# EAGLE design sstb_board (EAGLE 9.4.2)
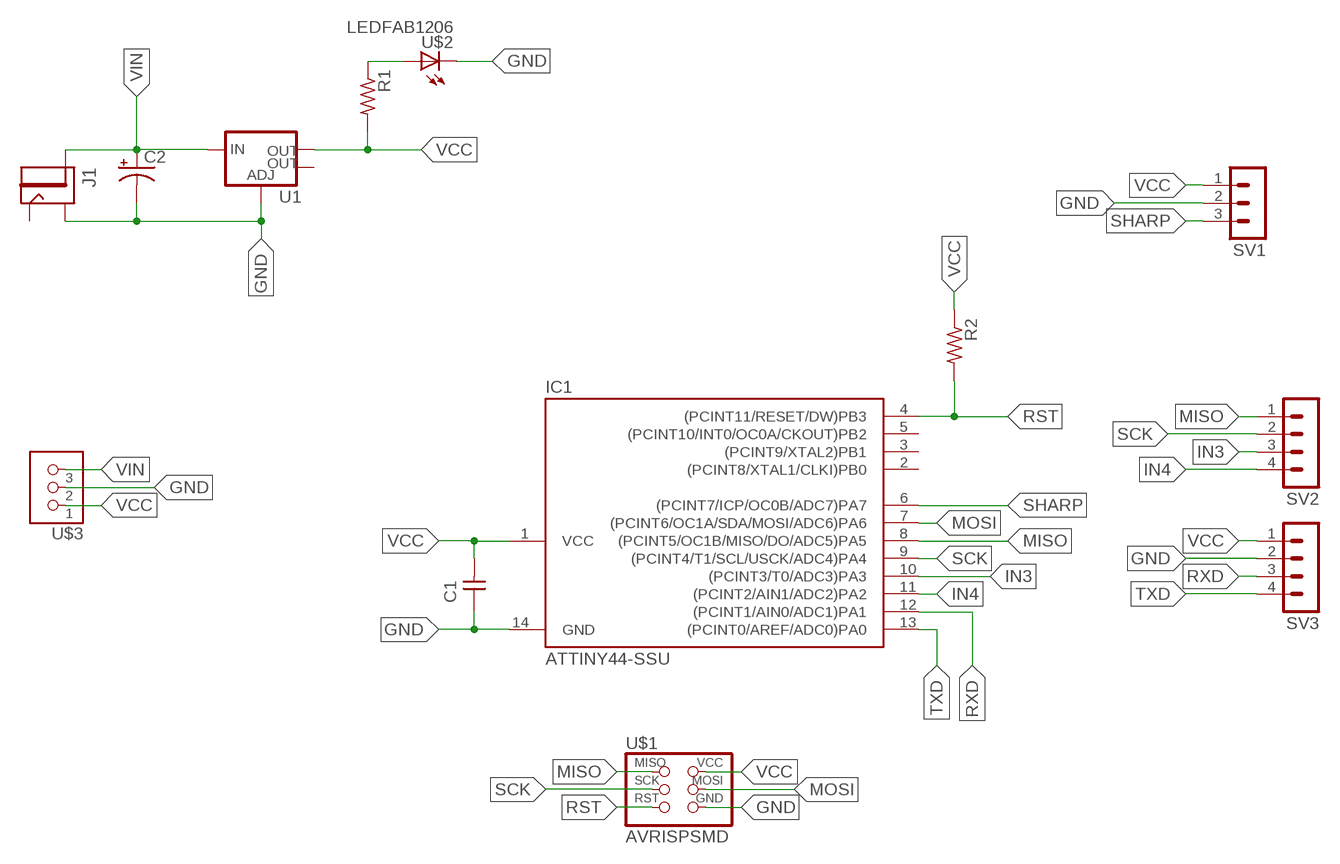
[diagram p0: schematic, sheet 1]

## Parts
C1  CAP-UNPOLARIZEDFAB  [C1206FAB]
C2  CPOL-USE5-8.5  [E5-8,5]
IC1  ATTINY44-SSU  [SOIC14]
J1  JACK2.1MM  [JACK_2.1MM]
R1  RES-US1206FAB  [R1206FAB]
R2  RES-US1206FAB  [R1206FAB]
SV1  MA03-1  [MA03-1]
SV2  MA04-1  [MA04-1]
SV3  MA04-1  [MA04-1]
U1  V_REG_LM1117SOT223  [SOT223]
U$1  AVRISPSMD  [2X03SMD]
U$2  LEDFAB1206  [LED1206FAB]
U$3  TERM-1X03'-FABLAB'  [ED555DS-3DS]

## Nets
GND: C1.1 C2.- IC1.14(GND) J1.SHUNT SV1.2 SV3.2 U1.1(ADJ) U$1.6(GND) U$2.2(C) U$3.2
IN3: IC1.10((PCINT3/T0/ADC3)PA3) SV2.3
IN4: IC1.11((PCINT2/AIN1/ADC2)PA2) SV2.4
MISO: IC1.8((PCINT5/OC1B/MISO/DO/ADC5)PA5) SV2.1 U$1.1(MISO)
MOSI: IC1.7((PCINT6/OC1A/SDA/MOSI/ADC6)PA6) U$1.4(MOSI)
N$21: R1.1 U$2.1(A)
RST: IC1.4((PCINT11/RESET/DW)PB3) R2.2 U$1.5(RST)
RXD: IC1.12((PCINT1/AIN0/ADC1)PA1) SV3.3
SCK: IC1.9((PCINT4/T1/SCL/USCK/ADC4)PA4) SV2.2 U$1.3(SCK)
SHARP: IC1.6((PCINT7/ICP/OC0B/ADC7)PA7) SV1.3
TXD: IC1.13((PCINT0/AREF/ADC0)PA0) SV3.4
VCC: C1.2 IC1.1(VCC) R1.2 R2.1 SV1.1 SV3.1 U1.2(OUT) U$1.2(VCC) U$3.1
VIN: C2.+ J1.PIN U1.3(IN) U$3.3
Unconnected: IC1.2((PCINT8/XTAL1/CLKI)PB0) IC1.3((PCINT9/XTAL2)PB1) IC1.5((PCINT10/INT0/OC0A/CKOUT)PB2) J1.CONTACT U1.4(OUT)

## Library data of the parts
C1 = fab:CAP-UNPOLARIZED
C2 = rcl:CPOL-US: POLARIZED CAPACITOR, American symbol; SPICEPREFIX: C
IC1 = fab:ATTINY44
J1 = fab:JACK
R1 R2 = fab:RES-US: Resistor (US Symbol)
SV1 = con-lstb:MA03-1: PIN HEADER; OC_FARNELL: unknown; OC_NEWARK: unknown
SV2 SV3 = con-lstb:MA04-1: PIN HEADER; OC_FARNELL: unknown; OC_NEWARK: unknown
U1 = fab:V_REG_LM1117: Voltage Regulator LM1117 Standard adjustable voltage regulator but in SMD form. Spark Fun Electronics SKU : COM-00595; PROD_ID: VREG-08170
U$1 = fab:AVRISP
U$2 = fab:LED: LED
U$3 = fab:TERM-1X03: 3.5mm terminal block, 3 positions ED555-3DS as found in the fablab inventory. Made by Zaerc.

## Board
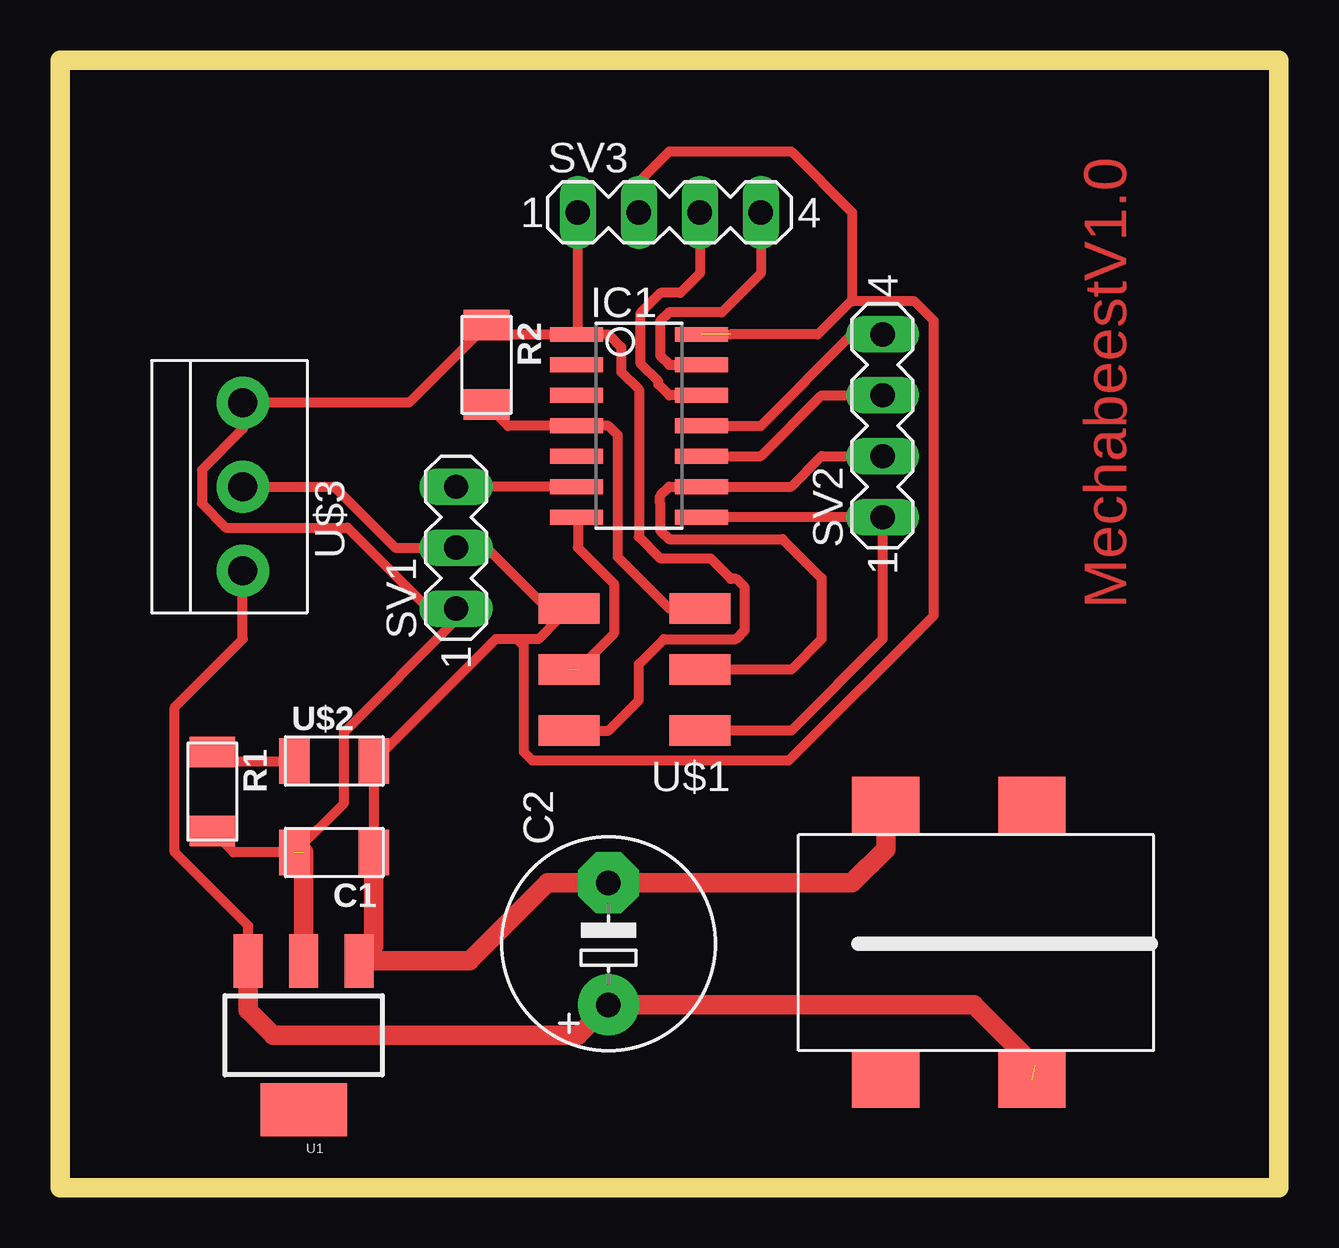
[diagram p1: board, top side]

Size 50.8 x 46.99 mm. Coordinates in mm from the lower left corner, seen from the top.
Outline: 1.27,0 2.54,0 50.8,0 50.8,46.99 0,46.99 0,0 1.27,0
Copper layers (1*16): Top 0.035mm / dielectric 1.5mm / Bottom 0.035mm
Design rules "default *": minimum track width 16mil, minimum drill 0.35mm, track to track 16mil, track to pad 16mil, pad to pad 16mil, via to via 16mil, smd to smd 16mil, copper to edge 16mil, drill to drill 16mil, minimum pad ring 10mil, minimum via ring 8mil, stop-mask expansion 4mil, vias tented up to drill 0mil, thermal gap 10mil

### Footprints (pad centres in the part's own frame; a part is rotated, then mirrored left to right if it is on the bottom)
C1206FAB = smd 1.27 x 1.905: 1 -1.651,0; 2 1.651,0
E5-8,5 = drill 1.016 pad 2.54: + -2.54,0 | drill 1.016 pad 2.54 octagon: - 2.54,0
SOIC14 = smd 0.61 x 2.21: 1 -3.81,-2.603; 2 -2.54,-2.603; 3 -1.27,-2.603; 4 0,-2.603; 5 1.27,-2.603; 6 2.54,-2.603; 7 3.81,-2.603; 8 3.81,2.603; 9 2.54,2.603; 10 1.27,2.603; 11 0,2.603; 12 -1.27,2.603; 13 -2.54,2.603; 14 -3.81,2.603
JACK_2.1MM = smd 2.388 x 2.794: CONTACT 5.766,-2.413; PIN -5.639,-2.413; PIN1 -5.639,3.683; SHUNT 5.766,3.683
R1206FAB = smd 1.27 x 1.905: 1 -1.651,0; 2 1.651,0
MA03-1 = drill 1.016 long: 1 -2.54,0; 2 0,0; 3 2.54,0
MA04-1 = drill 1.016 long: 1 -3.81,0; 2 -1.27,0; 3 1.27,0; 4 3.81,0
SOT223 = smd 1.219 x 2.235: 1 -2.311,-3.099; 2 0,-3.099; 3 2.311,-3.099 | smd 3.6 x 2.2: 4 0,3.099
2X03SMD = smd 2.54 x 1.27: 1 -2.54,2.54; 2 2.92,2.54; 3 -2.54,0; 4 2.92,0; 5 -2.54,-2.54; 6 2.92,-2.54
LED1206FAB = smd 1.27 x 1.905: 1 -1.651,0; 2 1.651,0
ED555DS-3DS = drill 1.2 pad 2.184: 1 -3.5,0; 2 0,0; 3 3.5,0

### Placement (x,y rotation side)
C1  11.43,13.97 180 top
C2  22.86,10.16 90 top
IC1  24.13,31.75 270 top
J1  38.1,10.16 90 top
R1  6.35,16.51 270 top
R2  17.78,34.29 270 top
SV1  16.51,26.67 90 top
SV2  34.29,31.75 90 top
SV3  25.4,40.64 0 top
U1  10.16,6.35 180 top
U$1  24.13,21.59 180 top
U$2  11.43,17.78 0 top
U$3  7.62,29.21 270 top

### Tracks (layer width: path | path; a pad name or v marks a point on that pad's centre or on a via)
GND  (1 unrouted)
  Top 0.406: C1.1 U$2.2 18.16,22.86 19.05,22.86 | U$1.6 20.77,23.69 | 20.77,23.69 19.94,22.86 19.05,22.86 | 20.77,23.69 17.78,26.67 SV1.2 13.97,26.67 11.43,29.21 U$3.2 | 33.02,36.93 35.62,36.93 36.42,36.13 36.42,23.84 30.38,17.8 19.69,17.8 19.33,18.16 19.33,22.58 19.05,22.86 | 33.02,36.93 32.96,36.93 31.59,35.56 27.94,35.56 | SV3.2 24.13,41.91 25.4,43.18 30.48,43.18 33.02,40.64 33.02,36.93
  Top 0.813: J1.SHUNT 34.42,14.1 33.02,12.7 C2.- 20.32,12.7 17.07,9.45 U1.1 13.08,10.06 C1.1
IN3
  Top 0.406: IC1.10 29.21,30.48 31.75,33.02 SV2.3
IN4
  Top 0.406: IC1.11 29.21,31.75 33.02,35.56 SV2.4
MISO
  Top 0.406: IC1.8 SV2.1 34.29,22.86 30.48,19.05 U$1.1
MOSI  (1 unrouted)
  Top 0.406: IC1.7 21.59,27.88 21.59,26.67 23.09,25.17 23.09,23.09 21.59,21.59
N$21
  Top 0.406: R1.1 6.73,17.78 U$2.1
RST
  Top 0.406: U$1.5 25.4,24.13 23.24,26.29 23.24,31.37 22.86,31.75 IC1.4 18.67,31.75 R2.2
RXD
  Top 0.406: SV3.3 26.67,38.1 25.86,37.29 25.04,37.29 24.21,36.45 24.21,34.33 24.94,33.6 24.94,33.48 25.4,33.02 IC1.12
SCK
  Top 0.406: SV2.2 31.75,30.48 30.48,29.21 IC1.9 25.4,29.21 25.02,28.83 25.02,28.5 25.02,27.94 25.02,27.38 25.38,27.03 30.12,27.03 31.75,25.4 31.75,22.86 30.48,21.59 U$1.3
SHARP
  Top 0.406: IC1.6 SV1.3
TXD
  Top 0.406: SV3.4 29.21,38.1 27.58,36.47 25.38,36.47 25.02,36.12 25.02,34.67 25.4,34.29 IC1.13
VCC  (1 unrouted)
  Top 0.406: R1.2 7.24,13.97 C1.2 11.84,16.03 11.84,18.98 16.51,23.66 SV1.1 15.36,24.13 11.98,27.51 6.91,27.51 5.92,28.51 5.92,29.91 7.62,31.62 U$3.1 14.55,32.71 R2.1 18.16,35.56 IC1.1 | U$1.2 22.86,19.05 24.13,20.32 24.13,21.82 25.17,22.86 28.17,22.86 28.55,23.24 28.55,25.02 28.19,25.38 27.96,25.38 27.13,26.21 25.04,26.21 24.13,27.12 24.13,33.26 23.39,34 23.39,35.03 22.86,35.56 IC1.1 | IC1.1 21.59,35.62 SV3.1
  Top 0.813: U1.2 10.16,13.97
VIN  (1 unrouted)
  Top 0.406: U1.3 7.85,10.91 4.79,13.97 4.79,20.03 7.62,22.86 U$3.3
  Top 0.813: 40.64,5.08 38.1,7.62 C2.+ 21.59,6.35 8.89,6.35 7.85,7.39 U1.3

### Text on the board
Top: MechabeestV1.0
